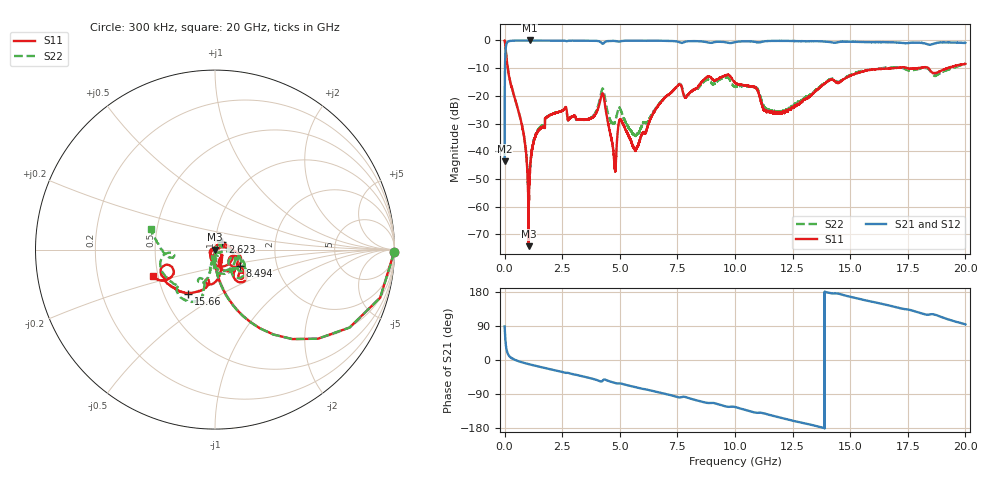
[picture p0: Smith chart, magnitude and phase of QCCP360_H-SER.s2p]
!{QCCP360}
!Johanson Technology Inc.
!www.johansontechnology.com
!Test Board Conditions:
!Substrate Type  RO4350B
!Substrate Thickness  20 mil
!Substrate Dk  3.66
!TL Type: GCPW
!TL Trace Width  36 mil
!TL Gap  12 mil
!Electrode orientation  Horizontal
!DUT TOPOLOGY	SERIES
!Mounting Pad LxW  26x36 mil
! Created Sat Jan  9 18:37:11 2021
# hz S ma R 50
! 2 Port Network Data from SP1.SP block
! freq  magS11  angS11  magS21  angS21  magS12  angS12  magS22  angS22
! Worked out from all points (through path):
!   20001 points, 300 kHz to 20 GHz, reference 50 ohm
!   highest |S21| = -0.01 dB at 1.092 GHz (marker M1); lowest = -43.7 dB at 300 kHz (marker M2)
!   group delay of S21, straight-line fit = 36.8 ps
!   lowest |S11| = -74.3 dB at 1.042 GHz (marker M3), VSWR 1.00, Z = 50 + j0.0111 ohm
!   |S11| at or under -10 dB: 136.1 MHz to 16.83 GHz (16.69 GHz wide, 197 % of centre); 17.49 GHz to 17.93 GHz (443.1 MHz wide, 2.5 % of centre); 18.4 GHz to 19.23 GHz (832.2 MHz wide, 4.42 % of centre)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
!   |S22| runs from -58.0 to 0.0 dB; largest |S21 - S12| = 0.017
!   S11 on the Smith chart (normalised r, x): 300 kHz: open; 2.623 GHz: 1.08, +0.10; 8.494 GHz: 1.29, -0.24; 15.66 GHz: 0.66, -0.35; 20 GHz: 0.47, -0.16
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300000  0.998 -0.7  0.006552 88.5  0.006605 89.0  1 -0.7
1.323e8  0.3243 -72.2  0.9437 17.5  0.9431 17.5  0.3257 -72.1
7.893e8  0.02484 -96.4  0.9974 -6.7  0.9979 -6.7  0.02503 -93.5
1.0423e9  0.0001932 145.1  0.9978 -10.8  0.9977 -10.8  0.00126 4.8
1.0923e9  0.003797 74.5  0.999 -11.7  0.9978 -11.6  0.004271 58.5
1.2163e9  0.01198 75.8  0.9967 -13.5  0.9977 -13.5  0.01247 68.6
1.4103e9  0.02171 73.1  0.9975 -16.3  0.9967 -16.3  0.02275 69.2
2.6233e9  0.06036 47.2  0.9873 -33.6  0.9874 -33.6  0.05945 52.5
3.3343e9  0.03741 52.1  0.9937 -42.4  0.9935 -42.4  0.03731 39.0
4.2583e9  0.1111 -45.4  0.8722 -54.4  0.872 -54.3  0.1352 -49.5
4.7753e9  0.0052 -145.2  0.9786 -60.3  0.9787 -60.3  0.03295 -74.2
5.0233e9  0.0374 -127.5  0.9649 -61.8  0.9647 -61.9  0.05739 -101.7
5.6993e9  0.01051 99.6  0.9925 -71.9  0.9917 -71.9  0.01921 -69.0
6.6673e9  0.06597 9.7  0.9901 -85.1  0.9881 -85.0  0.06822 -8.6
8.4943e9  0.165 -33.9  0.9658 -108.9  0.9647 -108.9  0.1533 -19.1
1.00003e10  0.1714 -52.9  0.9328 -124.1  0.9328 -124.1  0.1463 -47.8
1.08963e10  0.1401 -58.7  0.9404 -139.0  0.9398 -139.0  0.144 -69.5
1.17023e10  0.05063 -40.1  0.9824 -148.1  0.9823 -147.9  0.05296 -82.9
1.33343e10  0.1054 -72.1  0.9698 -171.4  0.9725 -171.4  0.1089 -103.8
1.56643e10  0.2869 -121.5  0.9347 157.6  0.9437 157.3  0.2866 -105.9
1.66673e10  0.311 -136.5  0.9286 144.1  0.9188 143.9  0.3249 -117.5
2e10  0.3786 -157.2  0.9021 93.9  0.8919 93.8  0.3787 162.0
